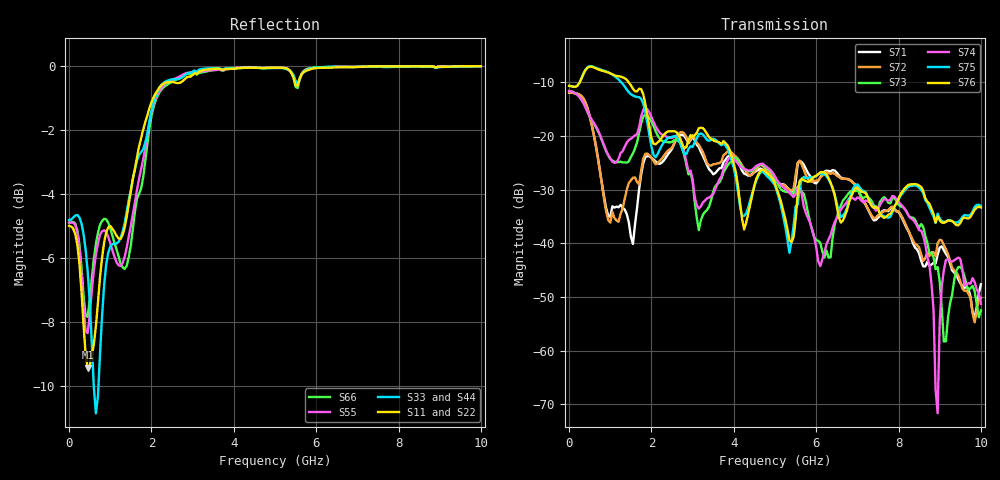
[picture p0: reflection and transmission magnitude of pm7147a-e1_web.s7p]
# GHz S DB R 50
! S-Parameters data
! Freq  dbS11  angS11  dbS12  angS12  dbS13  angS13  dbS14  angS14
!  dbS15  angS15  dbS16  angS16  dbS17  angS17  dbS21  angS21
!  dbS22  angS22  dbS23  angS23  dbS24  angS24  dbS25  angS25
!  dbS26  angS26  dbS27  angS27  dbS31  angS31  dbS32  angS32
!  dbS33  angS33  dbS34  angS34  dbS35  angS35  dbS36  angS36
!  dbS37  angS37  dbS41  angS41  dbS42  angS42  dbS43  angS43
!  dbS44  angS44  dbS45  angS45  dbS46  angS46  dbS47  angS47
!  dbS51  angS51  dbS52  angS52  dbS53  angS53  dbS54  angS54
!  dbS55  angS55  dbS56  angS56  dbS57  angS57  dbS61  angS61
!  dbS62  angS62  dbS63  angS63  dbS64  angS64  dbS65  angS65
!  dbS66  angS66  dbS67  angS67  dbS71  angS71  dbS72  angS72
!  dbS73  angS73  dbS74  angS74  dbS75  angS75  dbS76  angS76
!  dbS77  angS77
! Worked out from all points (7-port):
!   279 points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, 1 Hz to 10 GHz, reference 50 ohm
!   strongest paths, dB at 1 Hz, 7.943 MHz, 3.05 GHz, 6.55 GHz, 10 GHz:
!     S76: -10.6, -10.7, -19.8, -35.2, -33.3
!     S75: -10.6, -10.7, -21.1, -34.0, -33.0
!     S74: -11.6, -11.6, -31.4, -34.5, -51.3
!     S73: -11.6, -11.6, -32.3, -34.0, -52.5
!     S72: -11.9, -11.9, -20.4, -27.6, -50.1
!     S71: -11.9, -11.9, -20.8, -27.3, -47.6
!   lowest |S11| = -9.4 dB at 450 MHz (marker M1), VSWR 2.02, Z = 24.8 + j0.806 ohm
!   |S11| at or under -10 dB: nowhere
